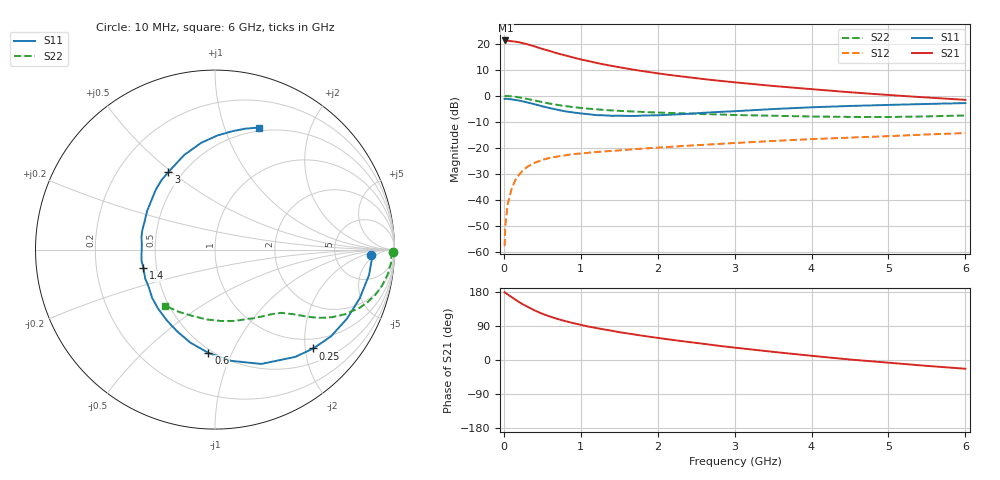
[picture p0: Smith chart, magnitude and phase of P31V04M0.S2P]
! SIEMENS Small Signal Semiconductors
! BFP181
! Si NPN RF Bipolar Junction Transistor in SOT143
! VCE = 1 V  IC = 4 mA
! Common Emitter S-Parameters:  March  1996
# GHz  S  MA  R  50
!  f  S11  S21  S12  S22
! GHz  MAG  ANG  MAG  ANG  MAG  ANG  MAG  ANG
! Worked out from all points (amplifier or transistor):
!   36 points, 10 MHz to 6 GHz, reference 50 ohm
!   highest |S21| = 21.2 dB at 20 MHz (marker M1)
!   |S21| within 3 dB of that: start of sweep to 475.9 MHz
!   unconditionally stable (mu >= 1): 1.604 GHz to end of sweep
!   at 250 MHz: K = 0.22, MSG = 24.4 dB, |S12| = -28.6 dB
!   at 1.4 GHz: K = 0.92, MSG = 16.3 dB, |S12| = -21.2 dB
!   at 6 GHz: K = 1.12, MAG = 4.3 dB, |S12| = -14.3 dB
!   S11 on the Smith chart (normalised r, x): 10 MHz: 13, -3; 250 MHz: 0.78, -2.17; 600 MHz: 0.47, -0.82; 1.4 GHz: 0.42, -0.11; 3 GHz: 0.42, +0.49; 6 GHz: 0.46, +1.31
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0.01  0.8675 -2.0  11.39 178.8  0.0013 89.1  0.9895 -0.7
0.02  0.8746 -4.0  11.48 177.6  0.0033 89.9  0.9832 -1.6
0.05  0.8699 -9.4  11.35 172.9  0.0083 87.6  0.984 -4.2
0.15  0.8299 -27.6  10.88 159.3  0.0242 74.2  0.9524 -12.1
0.2  0.807 -36.8  10.58 152.8  0.0308 70.0  0.9293 -15.6
0.25  0.7765 -45.2  10.15 146.6  0.037 65.2  0.9001 -18.9
0.3  0.7466 -53.2  9.764 141.4  0.0428 62.0  0.8701 -21.8
0.4  0.6871 -68.0  8.828 130.8  0.0517 55.5  0.8095 -26.4
0.5  0.626 -81.8  7.916 122.0  0.0586 50.6  0.7548 -29.9
0.6  0.5769 -93.6  7.202 114.6  0.0646 46.2  0.7055 -32.6
0.7  0.536 -104.9  6.46 108.2  0.0683 43.3  0.6648 -34.6
0.8  0.5016 -115.0  5.927 102.5  0.0719 41.1  0.6328 -36.1
0.9  0.4773 -124.1  5.421 97.5  0.076 39.2  0.6058 -37.4
1.1  0.4416 -142.5  4.619 88.2  0.0807 36.7  0.5639 -39.6
1.4  0.4119 -165.3  3.744 77.3  0.0874 34.2  0.5222 -42.7
1.8  0.4157 170.1  2.974 64.1  0.0966 32.8  0.4892 -46.9
2.2  0.435 150.5  2.451 52.8  0.1055 31.3  0.4646 -52.1
3  0.5042 121.0  1.808 32.7  0.1237 28.3  0.4269 -64.6
3.5  0.5545 108.0  1.539 21.5  0.1355 25.9  0.4128 -74.3
4.5  0.6359 88.8  1.165 1.3  0.1572 20.0  0.3921 -96.6
5.5  0.6947 75.9  0.924 -15.5  0.1806 14.9  0.401 -120.0
6  0.7221 70.3  0.833 -23.1  0.192 11.3  0.4179 -131.6
